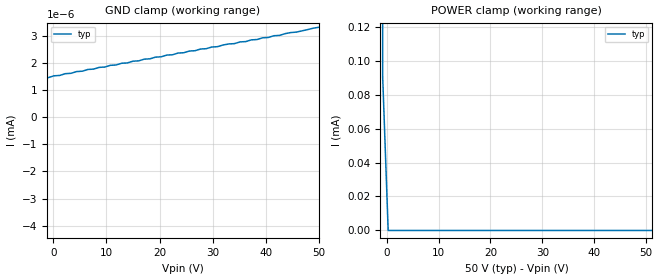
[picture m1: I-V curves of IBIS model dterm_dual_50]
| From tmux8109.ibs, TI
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| dterm_dual_50
[Model]   dterm_dual_50
Model_type   Terminator
|   typ   min   max
C_comp   4.014581e-12   NA   NA
[Voltage Range]   50   NA   NA
[Temperature Range]   27   NA   NA
[Power Clamp Reference]   50   NA   NA
[GND Clamp Reference]   0   NA   NA
[GND Clamp]
|   Voltage   I(typ)   I(min)   I(max)
-55V      -2.259A    NA         NA
-50.76V   -1.172mA   NA         NA
-49.7V    -653.5pA   NA         NA
-44.39V   -458.1pA   NA         NA
-30.61V   260.2pA    NA         NA
-13.64V   991.4pA    NA         NA
10.76V    1.906nA    NA         NA
11.82V    1.918nA    NA         NA
17.12V    2.132nA    NA         NA
18.18V    2.144nA    NA         NA
42.58V    3.008nA    NA         NA
50V       3.307nA    NA         NA
[POWER Clamp]
|   Voltage   I(typ)   I(min)   I(max)
-5V       744mA      NA         NA
-1.818V   145.4mA    NA         NA
-757.6mV  90.5uA     NA         NA
303mV     3.301nA    NA         NA
100V      -690.1pA   NA         NA
